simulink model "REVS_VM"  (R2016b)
settings: Solver=ode3  StartTime=REVS.sim_start_time_secs  StopTime=Inf  FixedStep=REVS.sim_step_time_secs  MaxStep=REVS.sim_step_time_secs  EnableMultiTasking=on
StopFcn:
  | postproc_datalog;
  | postproc_audit;
  | postproc_result;
model workspace (MATLAB code in the model file):
  other statements: REVS_setup_variants
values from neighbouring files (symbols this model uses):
  accessory = class_accessory_data    [class_test_data.m]
  battery = class_battery_data    [class_accessory_data.m]    (also in class_REVS_electric.m = class_REVS_battery)
  brake = struct(	'max_torque_Nm',[], 						'proportion_norm',1.0, 						'inertia_kgm2',0.0)    [class_REVS_drive_axle.m]
  engine = class_engine_data    [class_test_data.m]
  final_drive = struct(	'gear_ratio',[], 								'efficiency_norm',[], 								'inertia_kgm2',[] )    [class_REVS_drive_axle.m]
  gear = class_REVS_gearbox    [class_REVS_AT_transmission.m]
  tire = struct(	'radius_m',[], 						'rolling_resistance_coefficient',0, 						'vehicle_weight_norm',1.0,  						'wheel_slip_torque_Nm',[],  						'inertia_kgm2',0.0)    [class_REVS_drive_axle.m]
  torque_converter = class_REVS_torque_converter    [class_REVS_AT_transmission.m]
  transmission = class_transmission_data    [class_test_data.m]
  vehicle = class_vehicle_data    [class_test_data.m]
undefined symbols (not defined in the file or in its folder): alternator, ambient, controls, convert, DelayTimeSecs, drive_cycle, driver, electric, gear_strategy, InitialCondition, InitialValue, LoadSource, LookupStructure, MultiplyPosInputs, Normalize, NumPhases, REVS, SpeedSource, starter, tableshift, UpperSaturationLimit, Value, VerboseLevel, VerboseSignal
libraries: simulink x153
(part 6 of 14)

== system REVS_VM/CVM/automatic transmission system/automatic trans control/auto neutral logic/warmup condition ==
  bus : Inport
  Bus Creator : BusCreator  Inputs=10
  Bus Creator1 : BusCreator  Inputs=2
  Bus Selector : BusSelector  OutputSignals=var_sigs.var_sig1  OutputAsBus=on
  Data Type Conversion : DataTypeConversion  OutDataTypeStr=double
  Display : Display
  Fcn : Fcn
  Variable {1..10} (10 alike) : Constant  Value=nan
  out : Outport
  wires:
  Data Type Conversion/1 -> Fcn/1
  Bus Selector/1 -> Data Type Conversion/1, Display/1
  Bus Creator1/1 -> Bus Selector/1
  Fcn/1 -> out/1
  bus/1 -> Bus Creator1/1  "system_bus"
  Bus Creator/1 -> Bus Creator1/2  "var_sigs"
  Variable 1/1 -> Bus Creator/1  "var_sig1"
  Variable 2/1 -> Bus Creator/2  "var_sig2"
  Variable 3/1 -> Bus Creator/3  "var_sig3"
  Variable 4/1 -> Bus Creator/4  "var_sig4"
  Variable 5/1 -> Bus Creator/5  "var_sig5"
  Variable 6/1 -> Bus Creator/6  "var_sig6"
  Variable 7/1 -> Bus Creator/7  "var_sig7"
  Variable 8/1 -> Bus Creator/8  "var_sig8"
  Variable 9/1 -> Bus Creator/9  "var_sig9"
  Variable 10/1 -> Bus Creator/10  "var_sig10"

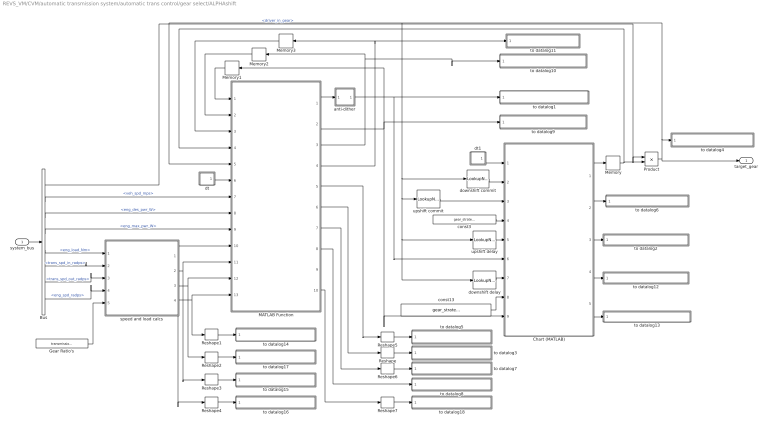
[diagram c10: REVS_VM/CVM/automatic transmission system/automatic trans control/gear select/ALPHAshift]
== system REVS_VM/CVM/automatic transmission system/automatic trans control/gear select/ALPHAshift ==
  system_bus : Inport
  Bus : BusSelector  OutputSignals=driver.driver_in_gear,vehicle.veh_spd_mps,powertrain.engine.eng_des_pwr_W,powertrain.engine.eng_max_pwr_W,powertrain.engine.eng_load_Nm,powertrain.trans.core.trans_spd_in_radps,powertrain.trans.core.trans_spd_out_radps,powertrain.engine.eng_spd_radps
  Chart (MATLAB) : Stateflow chart  TreatAsAtomicUnit=on
  Gear Ratio's : Constant  Value=transmission.gear.ratio  VectorParams1D=off
  MATLAB Function : MATLAB Function  TreatAsAtomicUnit=on
  Memory{,1..3} (4 alike) : Memory
  Product : Product
  Reshape{,1..7} (8 alike) : Reshape
  anti-dither : Subsystem
  const13 : Constant  Value=gear_strategy.disable_cost_saving_downshifts
  const3 : Constant  Value=gear_strategy.launch_gear_num
  downshift commit : LookupNDDirect  NumberOfTableDimensions=1  Table=gear_strategy.downshift_commit_secs
  downshift delay : LookupNDDirect  NumberOfTableDimensions=1  Table=gear_strategy.downshift_delay_secs
  dt : Subsystem
  dt1 : Subsystem
  speed and load calcs : Subsystem
  to datalog1 : Subsystem
  to datalog10 : Subsystem
  to datalog11 : Subsystem
  to datalog12 : Subsystem
  to datalog13 : Subsystem
  to datalog14 : Subsystem
  to datalog15 : Subsystem
  to datalog16 : Subsystem
  to datalog17 : Subsystem
  to datalog18 : Subsystem
  to datalog2 : Subsystem
  to datalog3 : Subsystem
  to datalog4 : Subsystem
  to datalog5 : Subsystem
  to datalog6 : Subsystem
  to datalog7 : Subsystem
  to datalog8 : Subsystem
  to datalog9 : Subsystem
  upshift commit : LookupNDDirect  NumberOfTableDimensions=1  Table=gear_strategy.upshift_commit_secs
  upshift delay : LookupNDDirect  NumberOfTableDimensions=1  Table=gear_strategy.upshift_delay_secs
  target_gear : Outport
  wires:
  MATLAB Function/10(kickdown_disability_code) -> Reshape7/1
  Reshape7/1 -> to datalog18/1(Var)
  Reshape2/1 -> to datalog17/1(Var)
  Chart (MATLAB)/5(in_gear_timer) -> to datalog13/1(Var)
  Chart (MATLAB)/4(shift_delay_timer) -> to datalog12/1(Var)
  speed and load calcs/1(gear_trq_Nm) -> Reshape4/1, MATLAB Function/10(gear_trq_Nm)
  Gear Ratio's/1 -> speed and load calcs/5(trans_gear_ratios)
  Bus/8 -> speed and load calcs/4(eng_spd_radps)  "<eng_spd_radps>"
  Bus/7 -> speed and load calcs/3(trans_spd_out_radps)  "<trans_spd_out_radps>"
  Bus/6 -> speed and load calcs/2(trans_spd_in_radps)  "<trans_spd_in_radps>"
  Bus/5 -> speed and load calcs/1(eng_load_Nm)  "<eng_load_Nm>"
  speed and load calcs/2(gear_spd_radps) -> Reshape3/1, MATLAB Function/11(gear_spd_radps)
  MATLAB Function/4(kickdown_ratio) -> to datalog11/1(Var), Memory3/1
  Memory3/1 -> MATLAB Function/3(kickdown_ratio_prev)
  Memory2/1 -> MATLAB Function/2(kickdown_timer_prev)
  MATLAB Function/3(kickdown_timer) -> Memory2/1, to datalog10/1(Var)
  Memory1/1 -> MATLAB Function/1(desired_shift_reason_prev)
  MATLAB Function/2(desired_shift_reason) -> to datalog9/1(Var), Memory1/1, Chart (MATLAB)/9(desired_shift_reason)
  const3/1 -> Chart (MATLAB)/4(launch_gear_num)
  const13/1 -> Chart (MATLAB)/8(legacy_downshift_mode)
  upshift delay/1 -> Chart (MATLAB)/5(upshift_delay_secs)
  downshift commit/1 -> Chart (MATLAB)/2(downshift_min_duration_secs)
  upshift commit/1 -> Chart (MATLAB)/3(upshift_min_duration_secs)
  downshift delay/1 -> Chart (MATLAB)/7(downshift_delay_secs)
  dt1/1(dt) -> Chart (MATLAB)/1(dt)
  Bus/1 -> Product/1  "<driver_in_gear>"
  Memory/1 -> MATLAB Function/4(command_gear_num), Product/2
  Bus/4 -> MATLAB Function/9(engine_max_pwr_W)  "<eng_max_pwr_W>"
  Bus/3 -> MATLAB Function/8(driver_des_pwr_W)  "<eng_des_pwr_W>"
  Chart (MATLAB)/2(previous_shift_type) -> to datalog6/1(Var)
  MATLAB Function/5(gear_available) -> Reshape5/1
  MATLAB Function/6(gear_disability_code) -> Reshape/1
  Chart (MATLAB)/3(shift_reason) -> to datalog2/1(Var)
  Product/1 -> MATLAB Function/5(current_gear_num), downshift commit/1, upshift commit/1, upshift delay/1, downshift delay/1, to datalog4/1(Var), target_gear/1
  system_bus/1 -> Bus/1
  speed and load calcs/3(gear_cost) -> MATLAB Function/12(gear_cost), Reshape2/1
  dt/1(dt) -> MATLAB Function/6(dt)
  Bus/2 -> MATLAB Function/7(vehicle_spd_mps)  "<veh_spd_mps>"
  Chart (MATLAB)/1(command_gear_num) -> Memory/1
  MATLAB Function/7(better_cost_gear) -> Reshape6/1
  MATLAB Function/8(min_cost_gear) -> to datalog8/1(Var)
  speed and load calcs/4(gear_avail_trq_Nm) -> Reshape1/1, MATLAB Function/13(gear_avail_trq_Nm)
  Reshape/1 -> to datalog3/1(Var)
  Reshape4/1 -> to datalog16/1(Var)
  Reshape3/1 -> to datalog15/1(Var)
  Reshape1/1 -> to datalog14/1(Var)
  anti-dither/1(out) -> to datalog1/1(Var), Chart (MATLAB)/6(desired_gear_num)
  MATLAB Function/1(desired_gear_num) -> anti-dither/1(raw)
  Reshape5/1 -> to datalog5/1(Var)
  Reshape6/1 -> to datalog7/1(Var)

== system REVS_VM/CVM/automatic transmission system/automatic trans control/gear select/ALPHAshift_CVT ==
  system_bus : Inport
  Bus Selector : BusSelector  OutputSignals=powertrain.trans.core.trans_spd_out_radps,driver.driver_in_gear,powertrain.engine.eng_des_pwr_W
  GR2SR : Fcn  Expr=1/u(1)
  MinMax : MinMax  Function=max  Inputs=2
  Product2 : Product  Inputs=**
  Product4 : Product  Inputs=*/
  SR Rate Limiter : RateLimiter  RisingSlewLimit=transmission.gear_strategy.speed_ratio_rise_rate_limit  FallingSlewLimit=-transmission.gear_strategy.speed_ratio_fall_rate_limit  SampleTimeMode=inherited
  SR2GR : Fcn  Expr=1/u(1)
  Saturation5 : Saturate  UpperLimit=max(transmission.gear.ratio)  LowerLimit=min(transmission.gear.ratio(2:end))
  eps : Saturate  UpperLimit=Inf  LowerLimit=eps
  min BSFC speed : Lookup_n-D  NumberOfTableDimensions=1  BreakpointsForDimension1=transmission.gear_strategy.min_bsfc_power_W  Table=transmission.gear_strategy.min_bsfc_speed_rapds  ExtrapMethod=Clip  InternalRulePriority=Speed  RndMeth=Simplest
  min speed table : Subsystem
  sat1 : Saturate  UpperLimit=2.48  LowerLimit=0.396
  sat2 : Saturate  UpperLimit=2.48  LowerLimit=0.396
  to datalog1 : Subsystem
  to datalog8 : Subsystem
  target_gear : Outport
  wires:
  MinMax/1 -> Product4/1, to datalog8/1(Var)
  min speed table/1(out) -> MinMax/2
  min BSFC speed/1 -> MinMax/1
  SR Rate Limiter/1 -> sat2/1
  Product2/1 -> GR2SR/1
  Bus Selector/2 -> Product2/1  "<driver_in_gear>"
  eps/1 -> Product4/2
  Saturation5/1 -> Product2/2
  Product4/1 -> Saturation5/1
  Bus Selector/3 -> min BSFC speed/1  "<eng_des_pwr_W>"
  Bus Selector/1 -> eps/1  "<trans_spd_out_radps>"
  system_bus/1 -> Bus Selector/1, min speed table/1(bus)
  SR2GR/1 -> target_gear/1, to datalog1/1(Var)
  sat2/1 -> SR2GR/1
  GR2SR/1 -> sat1/1
  sat1/1 -> SR Rate Limiter/1

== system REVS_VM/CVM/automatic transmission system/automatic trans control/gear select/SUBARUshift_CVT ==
  system_bus : Inport
  >= 1 : Saturate  UpperLimit=Inf  LowerLimit=1
  Bus Creator : BusCreator  Inputs=2
  Bus Creator1 : BusCreator  Inputs=2
  Bus Selector : BusSelector  OutputSignals=powertrain.trans.core.trans_spd_out_radps,driver.driver_in_gear
  Difference : simulink/Discrete/Difference  ICPrevInput=0.0  InputProcessing=Inherited  OutMin=[]  OutMax=[]  OutDataType=fixdt(1, 16)  OutScaling=2^-10  DoSatur=off
  Product : Product  Inputs=*/
  Product1 : Product  Inputs=*/
  Product2 : Product  Inputs=**
  Saturation : Saturate  UpperLimit=max(transmission.gear.ratio)  LowerLimit=min(transmission.gear.ratio(2:end))
  Saturation1 : Saturate  UpperLimit=max(transmission.gear.ratio)  LowerLimit=min(transmission.gear.ratio(2:end))
  Saturation2 : Saturate  UpperLimit=max(transmission.gear.ratio)  LowerLimit=min(transmission.gear.ratio(2:end))
  Switch : Switch  Criteria=u2 > Threshold
  downshift rate limit radps2 : Subsystem
  downshift time constant : Subsystem
  engine target radps : Subsystem
  eps : Saturate  UpperLimit=Inf  LowerLimit=eps
  target speed rate limiter : simulink/Discontinuities/Rate Limiter Dynamic
  upshift rate limit radps2 : Subsystem
  upshift time constant : Subsystem
  variable low pass filter : Subsystem
  target_gear : Outport
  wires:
  Product2/1 -> target_gear/1
  Saturation2/1 -> Product2/1  "cmd_ratio"
  Bus Selector/2 -> Product2/2  "<driver_in_gear>"
  engine target radps/1(out) -> >= 1/1
  variable low pass filter/1(out) -> Saturation2/1
  Switch/1 -> variable low pass filter/2(time const)
  Bus Creator1/1 -> downshift time constant/1(bus), upshift time constant/1(bus)
  upshift time constant/1(out) -> Switch/3
  downshift time constant/1(out) -> Switch/1
  Difference/1 -> Switch/2
  Saturation/1 -> variable low pass filter/1(in), Difference/1  "target_ratio"
  Bus Creator/1 -> downshift rate limit radps2/1(bus)
  Saturation1/1 -> Bus Creator/2  "desired_ratio"
  Product1/1 -> Saturation1/1
  >= 1/1 -> Product1/1, target speed rate limiter/2
  target speed rate limiter/1 -> Product/1, Bus Creator1/2  "desired_speed_radps"
  eps/1 -> Product1/2, Product/2
  upshift rate limit radps2/1(out) -> target speed rate limiter/3
  downshift rate limit radps2/1(out) -> target speed rate limiter/1
  Product/1 -> Saturation/1
  Bus Selector/1 -> eps/1  "<trans_spd_out_radps>"
  system_bus/1 -> upshift rate limit radps2/1(bus), Bus Selector/1, engine target radps/1(bus), Bus Creator/1, Bus Creator1/1

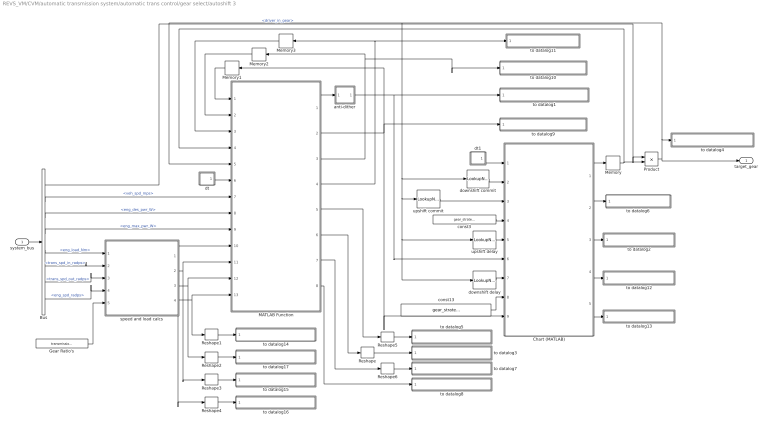
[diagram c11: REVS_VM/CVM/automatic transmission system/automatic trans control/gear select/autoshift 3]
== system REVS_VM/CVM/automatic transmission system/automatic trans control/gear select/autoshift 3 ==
  system_bus : Inport
  Bus : BusSelector  OutputSignals=driver.driver_in_gear,vehicle.veh_spd_mps,powertrain.engine.eng_des_pwr_W,powertrain.engine.eng_max_pwr_W,powertrain.engine.eng_load_Nm,powertrain.trans.core.trans_spd_in_radps,powertrain.trans.core.trans_spd_out_radps,powertrain.engine.eng_spd_radps
  Chart (MATLAB) : Stateflow chart  TreatAsAtomicUnit=on
  Gear Ratio's : Constant  Value=transmission.gear.ratio  VectorParams1D=off
  MATLAB Function : MATLAB Function  TreatAsAtomicUnit=on
  Memory{,1..3} (4 alike) : Memory
  Product : Product
  Reshape{,1..6} (7 alike) : Reshape
  anti-dither : Subsystem
  const13 : Constant  Value=gear_strategy.disable_cost_saving_downshifts
  const3 : Constant  Value=gear_strategy.launch_gear_num
  downshift commit : LookupNDDirect  NumberOfTableDimensions=1  Table=gear_strategy.downshift_commit_secs
  downshift delay : LookupNDDirect  NumberOfTableDimensions=1  Table=gear_strategy.downshift_delay_secs
  dt : Subsystem
  dt1 : Subsystem
  speed and load calcs : Subsystem
  to datalog1 : Subsystem
  to datalog10 : Subsystem
  to datalog11 : Subsystem
  to datalog12 : Subsystem
  to datalog13 : Subsystem
  to datalog14 : Subsystem
  to datalog15 : Subsystem
  to datalog16 : Subsystem
  to datalog17 : Subsystem
  to datalog2 : Subsystem
  to datalog3 : Subsystem
  to datalog4 : Subsystem
  to datalog5 : Subsystem
  to datalog6 : Subsystem
  to datalog7 : Subsystem
  to datalog8 : Subsystem
  to datalog9 : Subsystem
  upshift commit : LookupNDDirect  NumberOfTableDimensions=1  Table=gear_strategy.upshift_commit_secs
  upshift delay : LookupNDDirect  NumberOfTableDimensions=1  Table=gear_strategy.upshift_delay_secs
  target_gear : Outport
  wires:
  Reshape6/1 -> to datalog7/1(Var)
  Reshape5/1 -> to datalog5/1(Var)
  MATLAB Function/1(desired_gear_num) -> anti-dither/1(raw)
  anti-dither/1(out) -> to datalog1/1(Var), Chart (MATLAB)/6(desired_gear_num)
  Reshape1/1 -> to datalog14/1(Var)
  Reshape3/1 -> to datalog15/1(Var)
  Reshape4/1 -> to datalog16/1(Var)
  Reshape/1 -> to datalog3/1(Var)
  speed and load calcs/4(gear_avail_trq_Nm) -> MATLAB Function/13(gear_avail_trq_Nm), Reshape1/1
  MATLAB Function/8(min_cost_gear) -> to datalog8/1(Var)
  MATLAB Function/7(better_cost_gear) -> Reshape6/1
  Chart (MATLAB)/1(command_gear_num) -> Memory/1
  Bus/2 -> MATLAB Function/7(vehicle_spd_mps)  "<veh_spd_mps>"
  dt/1(dt) -> MATLAB Function/6(dt)
  speed and load calcs/3(gear_cost) -> Reshape2/1, MATLAB Function/12(gear_cost)
  system_bus/1 -> Bus/1
  Product/1 -> target_gear/1, to datalog4/1(Var), downshift delay/1, upshift delay/1, upshift commit/1, downshift commit/1, MATLAB Function/5(current_gear_num)
  Chart (MATLAB)/3(shift_reason) -> to datalog2/1(Var)
  MATLAB Function/6(gear_disability_code) -> Reshape/1
  MATLAB Function/5(gear_available) -> Reshape5/1
  Chart (MATLAB)/2(previous_shift_type) -> to datalog6/1(Var)
  Bus/3 -> MATLAB Function/8(driver_des_pwr_W)  "<eng_des_pwr_W>"
  Bus/4 -> MATLAB Function/9(engine_max_pwr_W)  "<eng_max_pwr_W>"
  Memory/1 -> Product/2, MATLAB Function/4(command_gear_num)
  Bus/1 -> Product/1  "<driver_in_gear>"
  dt1/1(dt) -> Chart (MATLAB)/1(dt)
  downshift delay/1 -> Chart (MATLAB)/7(downshift_delay_secs)
  upshift commit/1 -> Chart (MATLAB)/3(upshift_min_duration_secs)
  downshift commit/1 -> Chart (MATLAB)/2(downshift_min_duration_secs)
  upshift delay/1 -> Chart (MATLAB)/5(upshift_delay_secs)
  const13/1 -> Chart (MATLAB)/8(legacy_downshift_mode)
  const3/1 -> Chart (MATLAB)/4(launch_gear_num)
  MATLAB Function/2(desired_shift_reason) -> Memory1/1, Chart (MATLAB)/9(desired_shift_reason), to datalog9/1(Var)
  Memory1/1 -> MATLAB Function/1(desired_shift_reason_prev)
  MATLAB Function/3(kickdown_timer) -> to datalog10/1(Var), Memory2/1
  Memory2/1 -> MATLAB Function/2(kickdown_timer_prev)
  Memory3/1 -> MATLAB Function/3(kickdown_ratio_prev)
  MATLAB Function/4(kickdown_ratio) -> Memory3/1, to datalog11/1(Var)
  speed and load calcs/2(gear_spd_radps) -> MATLAB Function/11(gear_spd_radps), Reshape3/1
  Bus/5 -> speed and load calcs/1(eng_load_Nm)  "<eng_load_Nm>"
  Bus/6 -> speed and load calcs/2(trans_spd_in_radps)  "<trans_spd_in_radps>"
  Bus/7 -> speed and load calcs/3(trans_spd_out_radps)  "<trans_spd_out_radps>"
  Bus/8 -> speed and load calcs/4(eng_spd_radps)  "<eng_spd_radps>"
  Gear Ratio's/1 -> speed and load calcs/5(trans_gear_ratios)
  speed and load calcs/1(gear_trq_Nm) -> MATLAB Function/10(gear_trq_Nm), Reshape4/1
  Chart (MATLAB)/4(shift_delay_timer) -> to datalog12/1(Var)
  Chart (MATLAB)/5(in_gear_timer) -> to datalog13/1(Var)
  Reshape2/1 -> to datalog17/1(Var)

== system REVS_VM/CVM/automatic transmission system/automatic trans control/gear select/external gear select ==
  system_bus : Inport
  Bus Selector : BusSelector  OutputSignals=driver.cycle_pos_secs
  drive cycle : Lookup_n-D  NumberOfTableDimensions=1  BreakpointsForDimension1=transmission.gear_strategy.time_secs  IndexSearchMethod=Linear search  BeginIndexSearchUsingPreviousIndexResult=on  Table=transmission.gear_strategy.gear_num  InterpMethod=Flat  ExtrapMethod=Clip  UseLastTableValue=on  RndMeth=Simplest  MaximumIndicesForEachDimension=1e5
  target_gear : Outport
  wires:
  system_bus/1 -> Bus Selector/1
  Bus Selector/1 -> drive cycle/1  "<cycle_pos_secs>"
  drive cycle/1 -> target_gear/1

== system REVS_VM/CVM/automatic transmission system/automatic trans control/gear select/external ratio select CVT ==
  system_bus : Inport
  Bus Selector : BusSelector  OutputSignals=driver.cycle_pos_secs,driver.driver_in_gear
  CVT ratio : Lookup_n-D  NumberOfTableDimensions=1  BreakpointsForDimension1=gear_strategy.time_secs  IndexSearchMethod=Linear search  BeginIndexSearchUsingPreviousIndexResult=on  Table=gear_strategy.CVT_ratio  ExtrapMethod=Clip  UseLastTableValue=on  RndMeth=Simplest  MaximumIndicesForEachDimension=1e5
  Product2 : Product  Inputs=**
  Saturation3 : Saturate  UpperLimit=max(transmission.gear.ratio)  LowerLimit=min(transmission.gear.ratio(2:end))
  target_gear : Outport
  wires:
  Product2/1 -> target_gear/1
  Saturation3/1 -> Product2/1
  CVT ratio/1 -> Saturation3/1
  Bus Selector/1 -> CVT ratio/1  "<cycle_pos_secs>"
  system_bus/1 -> Bus Selector/1
  Bus Selector/2 -> Product2/2  "<driver_in_gear>"

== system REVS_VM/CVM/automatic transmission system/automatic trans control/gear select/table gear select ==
  system_bus : Inport
  Bus Selector : BusSelector  OutputSignals=driver.driver_in_gear
  Downshift : Lookup_n-D  BreakpointsForDimension1=tableshift.downshift_map_load  BreakpointsForDimension2=(1:size(tableshift.downshift_map_speed,2))-1  IndexSearchMethod=Linear search  BeginIndexSearchUsingPreviousIndexResult=on  Table=tableshift.downshift_map_speed  ExtrapMethod=Clip  DiagnosticForOutOfRangeInput=Error  UseLastTableValue=on  RndMeth=Simplest
  Downshift Delay : LookupNDDirect  NumberOfTableDimensions=1  Table=tableshift.downshift_delay_secs  DiagnosticForOutOfRangeInput=Error
  Memory1 : Memory  X0=1
  Product : Product
  Saturation : Saturate  UpperLimit=transmission.gear.number(end)  LowerLimit=0  ZeroCross=off
  Upshift : Lookup_n-D  BreakpointsForDimension1=tableshift.upshift_map_load  BreakpointsForDimension2=(1:size(tableshift.upshift_map_speed,2))-1  IndexSearchMethod=Linear search  BeginIndexSearchUsingPreviousIndexResult=on  Table=tableshift.upshift_map_speed  ExtrapMethod=Clip  DiagnosticForOutOfRangeInput=Error  UseLastTableValue=on  RndMeth=Simplest
  Upshift Delay : LookupNDDirect  NumberOfTableDimensions=1  Table=tableshift.upshift_delay_secs  DiagnosticForOutOfRangeInput=Error
  dt : Subsystem
  gear shifting : Stateflow chart  TreatAsAtomicUnit=on
  shift load select : Subsystem
  shift speed select : Subsystem
  target_gear : Outport
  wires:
  Saturation/1 -> target_gear/1
  Downshift Delay/1 -> gear shifting/6(downshift_delay_secs)
  Bus Selector/1 -> Product/2  "<driver_in_gear>"
  Product/1 -> Saturation/1
  shift speed select/1(spd) -> gear shifting/1(shift_spd)
  Downshift/1 -> gear shifting/5(downshift_spd)
  shift load select/1(load) -> Upshift/1, Downshift/1
  Upshift/1 -> gear shifting/4(upshift_spd)
  Upshift Delay/1 -> gear shifting/3(upshift_delay_secs)
  Memory1/1 -> Downshift Delay/1, Downshift/2, Upshift Delay/1, Upshift/2
  gear shifting/1(driver_gear) -> Memory1/1, Product/1
  system_bus/1 -> Bus Selector/1, shift speed select/1(system_bus), shift load select/1(system_bus)
  dt/1(dt) -> gear shifting/2(step_time)

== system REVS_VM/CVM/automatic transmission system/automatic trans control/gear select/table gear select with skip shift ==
  system_bus : Inport
  Bus Selector : BusSelector  OutputSignals=driver.driver_in_gear
  Compare To Constant : simulink/Logic and Bit Operations/Compare To Constant  relop=>  const=3.0  OutDataTypeStr=boolean  ZeroCross=off
  Constant : Constant
  Constant1 : Constant
  Down Shift Timer : Subsystem
  Downshift : Lookup_n-D  BreakpointsForDimension1=tableshift.downshift_map_load  BreakpointsForDimension2=(1:size(tableshift.downshift_map_speed,2))-1  IndexSearchMethod=Linear search  BeginIndexSearchUsingPreviousIndexResult=on  Table=tableshift.downshift_map_speed  ExtrapMethod=Clip  UseLastTableValue=on  RndMeth=Simplest
  Downshift Delay : LookupNDDirect  NumberOfTableDimensions=1  Table=tableshift.downshift_delay_secs
  Downshift Skip Pedal : LookupNDDirect  NumberOfTableDimensions=1  Table=tableshift.downshift_skip_pedal_pct
  Downshift Switch : Switch  Criteria=u2 ~= 0
  Logical Operator : Logic  AllPortsSameDT=off  OutDataTypeStr=boolean
  Memory4 : Memory  X0=1
  Product : Product
  Relational Operator : RelationalOperator  Operator=>  OutDataTypeStr=boolean  ZeroCross=off
  Relational Operator1 : RelationalOperator  Operator=<  OutDataTypeStr=boolean  ZeroCross=off
  Relational Operator2 : RelationalOperator  OutDataTypeStr=boolean  ZeroCross=off
  Relational Operator3 : RelationalOperator  Operator=>  OutDataTypeStr=boolean  ZeroCross=off
  Relational Operator4 : RelationalOperator  Operator=<=  OutDataTypeStr=boolean  ZeroCross=off
  Relational Operator5 : RelationalOperator  Operator=>  OutDataTypeStr=boolean  ZeroCross=off
  Saturation : Saturate  UpperLimit=inf  LowerLimit=1  ZeroCross=off
  Sum : Sum  Inputs=+++
  Sum1 : Sum  Inputs=+--
  Time Since Upshift : Subsystem
  Up Shift Timer : Subsystem
  Upshift : Lookup_n-D  BreakpointsForDimension1=tableshift.upshift_map_load  BreakpointsForDimension2=(1:size(tableshift.upshift_map_speed,2))-1  IndexSearchMethod=Linear search  BeginIndexSearchUsingPreviousIndexResult=on  Table=tableshift.upshift_map_speed  ExtrapMethod=Clip  UseLastTableValue=on  RndMeth=Simplest
  Upshift Delay : LookupNDDirect  NumberOfTableDimensions=1  Table=tableshift.upshift_delay_secs
  Upshift Skip Pedal : LookupNDDirect  NumberOfTableDimensions=1  Table=tableshift.upshift_skip_pedal_pct
  Upshift Switch : Switch  Criteria=u2 ~= 0
  load select : Subsystem
  speed select : Subsystem
  target_gear : Outport
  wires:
  Product/1 -> target_gear/1
  Bus Selector/1 -> Product/1  "<driver_in_gear>"
  system_bus/1 -> speed select/1(system_bus), load select/1(system_bus), Bus Selector/1
  Downshift Switch/1 -> Saturation/1
  Upshift Delay/1 -> Relational Operator3/2
  Upshift/1 -> Relational Operator/2
  load select/1(load) -> Upshift/1, Relational Operator2/1, Relational Operator4/1, Downshift/1
  Downshift/1 -> Relational Operator1/2
  speed select/1(spd) -> Relational Operator/1, Relational Operator1/1
  Relational Operator/1 -> Up Shift Timer/1(Bool)
  Relational Operator1/1 -> Down Shift Timer/1(Bool)
  Memory4/1 -> Upshift Skip Pedal/1, Upshift Delay/1, Upshift/2, Sum/3, Sum1/1, Downshift Skip Pedal/1, Downshift/2, Downshift Delay/1, Upshift Switch/3
  Downshift Delay/1 -> Relational Operator5/2
  Down Shift Timer/1(Timer) -> Relational Operator5/1
  Up Shift Timer/1(Timer) -> Relational Operator3/1
  Relational Operator3/1 -> Time Since Upshift/1(Bool), Upshift Switch/2
  Upshift Switch/1 -> Downshift Switch/3
  Relational Operator5/1 -> Logical Operator/2
  Upshift Skip Pedal/1 -> Relational Operator2/2
  Relational Operator2/1 -> Sum/2
  Constant/1 -> Sum/1
  Sum/1 -> Upshift Switch/1
  Constant1/1 -> Sum1/3
  Sum1/1 -> Downshift Switch/1
  Downshift Skip Pedal/1 -> Relational Operator4/2
  Relational Operator4/1 -> Sum1/2
  Saturation/1 -> Memory4/1, Product/2
  Logical Operator/1 -> Downshift Switch/2
  Time Since Upshift/1(Timer) -> Compare To Constant/1
  Compare To Constant/1 -> Logical Operator/1

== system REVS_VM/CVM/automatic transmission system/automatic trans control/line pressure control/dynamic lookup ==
  bus : Inport
  Bus Selector : BusSelector  OutputSignals=gb.gb_cmd_gear,gb_spd_in_radps,ctrl.gb_line_press_bar
  Lookup : Lookup_n-D  NumberOfTableDimensions=10  BreakpointsForDimension1=LookupStructure.axis_1.breakpoints  BreakpointsForDimension2=LookupStructure.axis_2.breakpoints  BreakpointsForDimension3=LookupStructure.axis_3.breakpoints  BreakpointsForDimension4=LookupStructure.axis_4.breakpoints  BreakpointsForDimension5=LookupStructure.axis_5.breakpoints  BreakpointsForDimension6=LookupStructure.axis_6.breakpoints  BreakpointsForDimension7=LookupStructure.axis_7.breakpoints  BreakpointsForDimension8=LookupStructure.axis_8.breakpoints  BreakpointsForDimension9=LookupStructure.axis_9.breakpoints  BreakpointsForDimension10=LookupStructure.axis_10.breakpoints  IndexSearchMethod=Linear search  BeginIndexSearchUsingPreviousIndexResult=on  Table=LookupStructure.table  DiagnosticForOutOfRangeInput=Warning  InternalRulePriority=Speed  RndMeth=Simplest  SupportTunableTableSize=on  MaximumIndicesForEachDimension=LookupStructure.table_size
  out : Outport
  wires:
  bus/1 -> Bus Selector/1
  Lookup/1 -> out/1

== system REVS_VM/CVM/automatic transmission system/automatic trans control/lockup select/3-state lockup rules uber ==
  gear_number : Inport
  system_bus : Inport  Port=2
  Bus Selector : BusSelector  OutputSignals=powertrain.trans.ctrl.gear_num
  Constant : Constant  Value=inf
  Constant1 : Constant  Value=transmission.tcc_strategy.upshift_slip_speed_radps
  Detect Decrease1 : simulink/Logic and Bit Operations/Detect Decrease  vinit=0.0  InputProcessing=Inherited  OutDataTypeStr=boolean
  Detect Increase1 : simulink/Logic and Bit Operations/Detect Increase  vinit=0.0  InputProcessing=Inherited  OutDataTypeStr=boolean
  MinMax : MinMax  Function=max  Inputs=3  ZeroCross=off
  Product : Product
  Product1 : Product
  Product2 : Product
  Rate Limiter : RateLimiter  RisingSlewLimit=transmission.tcc_strategy.disengage_rate_radps2  FallingSlewLimit=-transmission.tcc_strategy.engage_rate_radps2  InitialCondition=100
  Relay : Relay  OnSwitchValue=transmission.tcc_strategy.lockup_hysteresis_radps * 1.5  OffSwitchValue=transmission.tcc_strategy.lockup_hysteresis_radps * 0.5  ZeroCross=off
  Saturation : Saturate  UpperLimit=1000 * convert.rpm2radps  LowerLimit=0  ZeroCross=off
  Switch : Switch  Criteria=u2 > Threshold  Threshold=1000 * convert.rpm2radps
  downshift slip speed : Constant  Value=transmission.tcc_strategy.downshift_slip_speed_radps
  downshift timer : Subsystem
  target slip table : Subsystem
  upshift timer : Subsystem
  lockup_cmd : Outport
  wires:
  target slip table/1(out) -> Product2/2, Relay/1
  Relay/1 -> Product2/1
  Switch/1 -> lockup_cmd/1
  Saturation/1 -> Rate Limiter/1
  MinMax/1 -> Saturation/1, Switch/2
  Product1/1 -> MinMax/3
  Product/1 -> MinMax/2
  Constant1/1 -> Product1/2
  downshift slip speed/1 -> Product/2
  upshift timer/1(timer_bool) -> Product1/1
  Detect Increase1/1 -> upshift timer/1(trigger_bool)
  downshift timer/1(timer_bool) -> Product/1
  Detect Decrease1/1 -> downshift timer/1(trigger_bool)
  Product2/1 -> MinMax/1
  system_bus/1 -> Bus Selector/1, target slip table/1(bus)
  Bus Selector/1 -> Detect Decrease1/1, Detect Increase1/1  "<gear_num>"
  Rate Limiter/1 -> Switch/3
  Constant/1 -> Switch/1

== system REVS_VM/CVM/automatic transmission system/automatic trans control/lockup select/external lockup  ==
  gear_number : Inport
  system_bus : Inport  Port=2
  1-D Lookup Table : Lookup_n-D  NumberOfTableDimensions=1  BreakpointsForDimension1=transmission.tcc_strategy.time_sec  IndexSearchMethod=Linear search  BeginIndexSearchUsingPreviousIndexResult=on  Table=transmission.tcc_strategy.lock_up  InterpMethod=Flat  ExtrapMethod=Clip  InternalRulePriority=Speed  RndMeth=Simplest
  Bus Selector : BusSelector  OutputSignals=driver.cycle_pos_secs
  lockup_cmd : Outport
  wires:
  1-D Lookup Table/1 -> lockup_cmd/1  "tcc_lock_up_cmd"
  system_bus/1 -> Bus Selector/1
  Bus Selector/1 -> 1-D Lookup Table/1  "<cycle_pos_secs>"

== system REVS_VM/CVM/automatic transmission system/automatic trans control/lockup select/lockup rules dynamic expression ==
  gear_number : Inport
  system_bus : Inport  Port=2
  Compare To Constant : simulink/Logic and Bit Operations/Compare To Constant  relop=>=  const=transmission.torque_converter.always_lock_gear  OutDataTypeStr=boolean  ZeroCross=off
  Compare To Constant6 : simulink/Logic and Bit Operations/Compare To Constant  relop=>  const=transmission.torque_converter.always_unlock_gear  OutDataTypeStr=boolean  ZeroCross=off
  Data Type Conversion : DataTypeConversion
  Detect Decrease : simulink/Logic and Bit Operations/Detect Decrease  vinit=0.0  InputProcessing=Inherited  OutDataTypeStr=boolean
  Detect Increase : simulink/Logic and Bit Operations/Detect Increase  vinit=0.0  InputProcessing=Inherited  OutDataTypeStr=boolean
  Logical Operator1 : Logic  AllPortsSameDT=off  OutDataTypeStr=boolean
  Logical Operator2 : Logic  Operator=NAND  AllPortsSameDT=off  OutDataTypeStr=boolean
  Logical Operator3 : Logic  Operator=NOT  AllPortsSameDT=off  OutDataTypeStr=boolean
  Logical Operator6 : Logic  Operator=NAND  AllPortsSameDT=off  OutDataTypeStr=boolean
  Logical Operator8 : Logic  Operator=OR  Inputs=3  AllPortsSameDT=off  OutDataTypeStr=boolean
  Logical Operator9 : Logic  Inputs=5  AllPortsSameDT=off  OutDataTypeStr=boolean
  Memory : Memory
  Relational Operator : RelationalOperator  Operator=>  OutDataTypeStr=boolean  ZeroCross=off
  boolean integrator : Subsystem
  const1 : Constant  Value=transmission.torque_converter.lockup_allowed
  const3 : Constant  Value=transmission.torque_converter.lockup_delay_secs
  downshift unlock criteria : Subsystem
  lockup equation : Subsystem
  unlock equation : Subsystem
  upshift unlock criteria : Subsystem
  lockup_cmd : Outport
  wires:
  Memory/1 -> Logical Operator1/2
  Logical Operator3/1 -> Logical Operator1/1
  Logical Operator1/1 -> Logical Operator8/3
  upshift unlock criteria/1(out) -> Logical Operator2/1
  downshift unlock criteria/1(out) -> Logical Operator6/1
  unlock equation/1(out) -> Logical Operator3/1
  Compare To Constant/1 -> Logical Operator8/1
  Data Type Conversion/1 -> lockup_cmd/1, Memory/1  "tcc_lockup_cmd_bool"
  Relational Operator/1 -> Data Type Conversion/1
  const1/1 -> Logical Operator9/1
  boolean integrator/1(out) -> Relational Operator/1
  gear_number/1 -> Detect Decrease/1, Detect Increase/1, Compare To Constant/1, Compare To Constant6/1
  lockup equation/1(out) -> Logical Operator8/2
  Detect Decrease/1 -> Logical Operator6/2
  const3/1 -> Relational Operator/2
  Compare To Constant6/1 -> Logical Operator9/2
  Logical Operator8/1 -> Logical Operator9/5
  Logical Operator9/1 -> boolean integrator/1(bool)
  system_bus/1 -> lockup equation/1(bus), downshift unlock criteria/1(bus), upshift unlock criteria/1(bus), unlock equation/1(bus)
  Detect Increase/1 -> Logical Operator2/2
  Logical Operator2/1 -> Logical Operator9/4
  Logical Operator6/1 -> Logical Operator9/3

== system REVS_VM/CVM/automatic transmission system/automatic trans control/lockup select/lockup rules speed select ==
  gear_number : Inport
  system_bus : Inport  Port=2
  Compare To Constant : simulink/Logic and Bit Operations/Compare To Constant  relop=>=  const=transmission.torque_converter.always_lock_gear  OutDataTypeStr=boolean  ZeroCross=off
  Compare To Constant1 : simulink/Logic and Bit Operations/Compare To Constant  relop=>  const=transmission.torque_converter.lockup_speed  OutDataTypeStr=boolean  ZeroCross=off
  Compare To Constant2 : simulink/Logic and Bit Operations/Compare To Constant  relop=<  const=transmission.torque_converter.unlock_speed  OutDataTypeStr=boolean  ZeroCross=off
  Compare To Constant6 : simulink/Logic and Bit Operations/Compare To Constant  relop=>  const=transmission.torque_converter.always_unlock_gear  OutDataTypeStr=boolean  ZeroCross=off
  Data Type Conversion : DataTypeConversion
  Detect Decrease : simulink/Logic and Bit Operations/Detect Decrease  vinit=0.0  InputProcessing=Inherited  OutDataTypeStr=boolean
  Detect Increase : simulink/Logic and Bit Operations/Detect Increase  vinit=0.0  InputProcessing=Inherited  OutDataTypeStr=boolean
  Latch : Subsystem
  Logical Operator2 : Logic  Operator=NAND  AllPortsSameDT=off  OutDataTypeStr=boolean
  Logical Operator6 : Logic  Operator=NAND  AllPortsSameDT=off  OutDataTypeStr=boolean
  Logical Operator8 : Logic  Operator=OR  AllPortsSameDT=off  OutDataTypeStr=boolean
  Logical Operator9 : Logic  Inputs=5  AllPortsSameDT=off  OutDataTypeStr=boolean
  Relational Operator : RelationalOperator  Operator=>  OutDataTypeStr=boolean  ZeroCross=off
  boolean integrator : Subsystem
  const1 : Constant  Value=transmission.torque_converter.lockup_allowed
  const2 : Constant  Value=transmission.torque_converter.unlock_downshift_bool
  const3 : Constant  Value=transmission.torque_converter.lockup_delay_secs
  const4 : Constant  Value=transmission.torque_converter.unlock_upshift_bool
  lockup speed select : Subsystem
  lockup_cmd : Outport
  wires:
  lockup speed select/1(spd) -> Compare To Constant1/1, Compare To Constant2/1
  Compare To Constant2/1 -> Latch/2(Off)
  Compare To Constant/1 -> Logical Operator8/1
  Data Type Conversion/1 -> lockup_cmd/1  "tcc_lockup_cmd_bool"
  Relational Operator/1 -> Data Type Conversion/1
  const1/1 -> Logical Operator9/1
  boolean integrator/1(out) -> Relational Operator/1
  gear_number/1 -> Detect Increase/1, Compare To Constant/1, Detect Decrease/1, Compare To Constant6/1
  Latch/1(State) -> Logical Operator8/2
  Compare To Constant1/1 -> Latch/1(On)
  Detect Decrease/1 -> Logical Operator6/2
  const3/1 -> Relational Operator/2
  const2/1 -> Logical Operator6/1
  Compare To Constant6/1 -> Logical Operator9/2
  Logical Operator8/1 -> Logical Operator9/5
  Logical Operator9/1 -> boolean integrator/1(bool)
  system_bus/1 -> lockup speed select/1(system_bus)
  const4/1 -> Logical Operator2/1
  Detect Increase/1 -> Logical Operator2/2
  Logical Operator2/1 -> Logical Operator9/4
  Logical Operator6/1 -> Logical Operator9/3

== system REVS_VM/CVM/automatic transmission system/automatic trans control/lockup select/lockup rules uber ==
  gear_number : Inport
  system_bus : Inport  Port=2
  Bus Creator1 : BusCreator  Inputs=3
  Data Type Conversion : DataTypeConversion
  Detect Decrease : simulink/Logic and Bit Operations/Detect Decrease  vinit=0.0  InputProcessing=Inherited  OutDataTypeStr=boolean
  Detect Increase : simulink/Logic and Bit Operations/Detect Increase  vinit=0.0  InputProcessing=Inherited  OutDataTypeStr=boolean
  Logical Operator2 : Logic  Operator=NAND  AllPortsSameDT=off  OutDataTypeStr=boolean
  Logical Operator3 : Logic  Operator=NOT  AllPortsSameDT=off  OutDataTypeStr=boolean
  Logical Operator6 : Logic  Operator=NAND  AllPortsSameDT=off  OutDataTypeStr=boolean
  Logical Operator8 : Logic  Operator=OR  AllPortsSameDT=off  OutDataTypeStr=boolean
  Logical Operator9 : Logic  Inputs=5  AllPortsSameDT=off  OutDataTypeStr=boolean
  Memory : Memory
  Relational Operator : RelationalOperator  Operator=>  OutDataTypeStr=boolean  ZeroCross=off
  boolean integrator : Subsystem
  const1 : Constant  Value=transmission.tcc_strategy.lockup_allowed
  const3 : Constant  Value=transmission.tcc_strategy.lockup_delay_secs
  downshift unlock criteria : Subsystem
  lockup criteria : Subsystem
  lockup table : Subsystem
  unlock criteria : Subsystem
  unlock table : Subsystem
  upshift unlock criteria : Subsystem
  lockup_cmd : Outport
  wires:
  Memory/1 -> Logical Operator8/1
  lockup criteria/1(out) -> Logical Operator8/2
  unlock table/1(out) -> Bus Creator1/2  "table_unlock_spd"
  Bus Creator1/1 -> unlock criteria/1(bus), lockup criteria/1(bus)
  lockup table/1(out) -> Bus Creator1/1  "table_lock_spd"
  Logical Operator3/1 -> Logical Operator9/5
  upshift unlock criteria/1(out) -> Logical Operator2/1
  downshift unlock criteria/1(out) -> Logical Operator6/1
  unlock criteria/1(out) -> Logical Operator3/1
  Data Type Conversion/1 -> Memory/1, lockup_cmd/1  "tcc_lockup_cmd_bool"
  Relational Operator/1 -> Data Type Conversion/1
  const1/1 -> Logical Operator9/1
  boolean integrator/1(out) -> Relational Operator/1
  gear_number/1 -> Detect Decrease/1, Detect Increase/1
  Detect Decrease/1 -> Logical Operator6/2
  const3/1 -> Relational Operator/2
  Logical Operator8/1 -> Logical Operator9/4
  Logical Operator9/1 -> boolean integrator/1(bool)
  system_bus/1 -> downshift unlock criteria/1(bus), upshift unlock criteria/1(bus), lockup table/1(bus), unlock table/1(bus), Bus Creator1/3  "system_bus"
  Detect Increase/1 -> Logical Operator2/2
  Logical Operator2/1 -> Logical Operator9/3
  Logical Operator6/1 -> Logical Operator9/2

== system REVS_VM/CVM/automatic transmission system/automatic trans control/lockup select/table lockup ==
  gear_number : Inport
  system_bus : Inport  Port=2
  const : Constant  Value=transmission.tcc_strategy.lockup_allowed
  const2 : Constant  Value=transmission.tcc_strategy.lockup_delay_secs
  dt : Subsystem
  "lock map " : Lookup_n-D  BreakpointsForDimension1=transmission.tcc_strategy.lock_map_load  BreakpointsForDimension2=transmission.gear.number(2:end)  Table=transmission.tcc_strategy.lock_map_speed  RndMeth=Simplest
  lockup load select : Subsystem
  lockup speed select : Subsystem
  tcc lockup : Stateflow chart  TreatAsAtomicUnit=on
  "unlock map " : Lookup_n-D  BreakpointsForDimension1=transmission.tcc_strategy.unlock_map_load  BreakpointsForDimension2=transmission.gear.number(2:end)  Table=transmission.tcc_strategy.unlock_map_speed  RndMeth=Simplest
  lockup_cmd : Outport
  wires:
  gear_number/1 -> "unlock map "/2, "lock map "/2
  system_bus/1 -> lockup speed select/1(system_bus), lockup load select/1(system_bus)
  const2/1 -> tcc lockup/6(lockup_delay_secs)
  lockup load select/1(load) -> "lock map "/1, "unlock map "/1
  const/1 -> tcc lockup/5(lockup_allowed)
  tcc lockup/1(tcc_lockup) -> lockup_cmd/1  "tcc_lockup_cmd_bool"
  "lock map "/1 -> tcc lockup/3(lockup_spd)
  "unlock map "/1 -> tcc lockup/4(release_spd)
  lockup speed select/1(spd) -> tcc lockup/1(lock_spd)
  dt/1(dt) -> tcc lockup/2(step_time)

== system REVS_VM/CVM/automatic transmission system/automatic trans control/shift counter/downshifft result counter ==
  in : Inport
  Data Type Conversion : DataTypeConversion  OutDataTypeStr=double
  Phase Memory : Memory
  Phase To Workspace : ToWorkspace  VariableName=result__phase_num_downshifts  SampleTime=-1
  Product : Product
  Sum : Sum  Inputs=|++
  Sum1 : Sum  Inputs=|++
  Total Memory : Memory
  Total To Workspace : ToWorkspace  VariableName=result__total_num_downshifts  SampleTime=-1
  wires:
  Data Type Conversion/1 -> Product/2, Sum1/1
  Sum1/1 -> Total Memory/1
  Sum/1 -> Phase Memory/1
  in/1 -> Data Type Conversion/1
  Total Memory/1 -> Sum1/2, Total To Workspace/1
  Product/1 -> Sum/1
  [REVS_phase_flag] -> Product/1
  Phase Memory/1 -> Phase To Workspace/1, Sum/2

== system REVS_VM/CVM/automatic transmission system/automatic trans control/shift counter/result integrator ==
  in : Inport
  Data Type Conversion : DataTypeConversion  OutDataTypeStr=double
  Integrator1 : Integrator  UpperSaturationLimit=Inf  LowerSaturationLimit=0  ZeroCross=off
  Integrator2 : Integrator  UpperSaturationLimit=Inf  LowerSaturationLimit=0  ZeroCross=off
  Phase To Workspace : ToWorkspace  VariableName=result__phase_gear_time_secs  SampleTime=-1
  Product1 : Product  Multiplication=Matrix(*)
  Reshape : Reshape
  Total To Workspace : ToWorkspace  VariableName=result__total_gear_time_secs  SampleTime=-1
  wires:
  Reshape/1 -> Integrator1/1, Product1/1
  Data Type Conversion/1 -> Reshape/1
  Integrator2/1 -> Phase To Workspace/1
  [REVS_phase_flag] -> Product1/2
  Product1/1 -> Integrator2/1
  Integrator1/1 -> Total To Workspace/1
  in/1 -> Data Type Conversion/1

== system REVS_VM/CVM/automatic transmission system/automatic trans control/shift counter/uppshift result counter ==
  in : Inport
  Data Type Conversion : DataTypeConversion  OutDataTypeStr=double
  Phase Memory : Memory
  Phase To Workspace : ToWorkspace  VariableName=result__phase_num_upshifts  SampleTime=-1
  Product : Product
  Sum : Sum  Inputs=|++
  Sum1 : Sum  Inputs=|++
  Total Memory : Memory
  Total To Workspace : ToWorkspace  VariableName=result__total_num_upshifts  SampleTime=-1
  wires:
  Data Type Conversion/1 -> Product/2, Sum1/1
  Sum1/1 -> Total Memory/1
  Sum/1 -> Phase Memory/1
  in/1 -> Data Type Conversion/1
  Total Memory/1 -> Sum1/2, Total To Workspace/1
  Product/1 -> Sum/1
  [REVS_phase_flag] -> Product/1
  Phase Memory/1 -> Phase To Workspace/1, Sum/2

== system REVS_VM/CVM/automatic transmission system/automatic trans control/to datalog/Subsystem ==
  In1 : Inport
  Enable : EnablePort
  To Workspace : ToWorkspace  VariableName=datalog__transmission__torque_converter_clutch_command_norm  SampleTime=-1
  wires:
  In1/1 -> To Workspace/1

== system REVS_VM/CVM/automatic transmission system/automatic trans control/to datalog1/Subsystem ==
  In1 : Inport
  Enable : EnablePort
  To Workspace : ToWorkspace  VariableName=datalog__transmission__selected_gear_num  SampleTime=-1
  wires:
  In1/1 -> To Workspace/1

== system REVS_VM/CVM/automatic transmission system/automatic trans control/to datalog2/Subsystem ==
  In1 : Inport
  Enable : EnablePort
  To Workspace : ToWorkspace  VariableName=datalog__transmission__command_line_pressure_bar  SampleTime=-1
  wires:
  In1/1 -> To Workspace/1

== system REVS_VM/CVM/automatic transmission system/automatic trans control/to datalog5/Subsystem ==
  In1 : Inport
  Enable : EnablePort
  To Workspace : ToWorkspace  VariableName=datalog__transmission__current_gear  SampleTime=-1
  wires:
  In1/1 -> To Workspace/1

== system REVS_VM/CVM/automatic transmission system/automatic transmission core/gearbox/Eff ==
  Efficiency : Inport
  Input : Inport  Port=2
  Math Function : Math  Operator=reciprocal
  Product1 : Product
  Switch : Switch  ZeroCross=off
  Output : Outport
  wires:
  Math Function/1 -> Switch/3
  Product1/1 -> Output/1
  Input/1 -> Product1/2, Switch/2
  Efficiency/1 -> Switch/1, Math Function/1
  Switch/1 -> Product1/1

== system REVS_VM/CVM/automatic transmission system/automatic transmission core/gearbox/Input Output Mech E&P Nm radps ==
  trq_in_Nm : Inport
  spd_in_radps : Inport  Port=2
  iner_in_kgm2 : Inport  Port=3
  trq_out_Nm : Inport  Port=4
  spd_out_radps : Inport  Port=5
  iner_out_kgm2 : Inport  Port=6
  Compare To Constant : simulink/Logic and Bit Operations/Compare To Constant  relop=>=  const=1  OutDataTypeStr=boolean
  Constant : Constant  Value=VerboseSignal
  Subsystem : Subsystem
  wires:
  trq_in_Nm/1 -> Subsystem/1(trq_in_Nm)
  spd_in_radps/1 -> Subsystem/2(spd_in_radps)
  iner_in_kgm2/1 -> Subsystem/3(iner_in_kgm2)
  trq_out_Nm/1 -> Subsystem/4(trq_out_Nm)
  spd_out_radps/1 -> Subsystem/5(spd_out_radps)
  iner_out_kgm2/1 -> Subsystem/6(iner_out_kgm2)
  Compare To Constant/1 -> Subsystem/Enable
  Constant/1 -> Compare To Constant/1

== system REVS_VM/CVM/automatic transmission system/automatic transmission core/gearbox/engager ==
  tgt_gear_num : Inport
  Compare To Constant1 : simulink/Logic and Bit Operations/Compare To Constant  relop=>  const=0  OutDataTypeStr=boolean  ZeroCross=off
  Compare To Constant2 : simulink/Logic and Bit Operations/Compare To Constant  relop=~=  const=0  OutDataTypeStr=boolean
  Compare To Constant3 : simulink/Logic and Bit Operations/Compare To Constant  relop=>=  const=1  OutDataTypeStr=boolean  ZeroCross=off
  Compare To Constant4 : simulink/Logic and Bit Operations/Compare To Constant  relop=~=  const=1  OutDataTypeStr=boolean  ZeroCross=off
  Compare To Constant5 : simulink/Logic and Bit Operations/Compare To Constant  relop=~=  const=0  OutDataTypeStr=boolean
  Constant1 : Constant  Value=gear.number
  Constant2 : Constant  Value=gear.type == enum_transmission_type.CVT
  Data Type Conversion : DataTypeConversion  OutDataTypeStr=double
  IC : InitialCondition  Value=0
  Logical Operator : Logic  Operator=OR  AllPortsSameDT=off  OutDataTypeStr=boolean
  Logical Operator1 : Logic  Operator=OR  Inputs=1  AllPortsSameDT=off  OutDataTypeStr=boolean
  Logical Operator2 : Logic  Inputs=3  AllPortsSameDT=off  OutDataTypeStr=boolean
  Memory1 : Memory  X0=gear.number(2)
  Memory2 : Memory  X0=gear.number(2)
  Product : Product
  Product1 : Product
  Rate Limiter : RateLimiter  RisingSlewLimit=1/gear.shift_duration_secs  FallingSlewLimit=-inf  InitialCondition=1
  Relational Operator : RelationalOperator  Operator===  OutDataTypeStr=boolean
  Relational Operator2 : RelationalOperator  Operator===  OutDataTypeStr=boolean
  Saturation : Saturate  UpperLimit=1  LowerLimit=0  ZeroCross=off
  Saturation1 : Saturate  UpperLimit=1 - 0.10 * (gear.type == enum_transmission_type.CVT)  LowerLimit=eps + 0.89 * (gear.type == enum_transmission_type.CVT)  ZeroCross=off
  Switch : Switch  Criteria=u2 > Threshold
  Switch1 : Switch  Criteria=u2 > Threshold
  to datalog with base name : Subsystem
  to datalog with base name1 : Subsystem
  to datalog with base name2 : Subsystem
  engage : Outport
  curr_gear_num : Outport  Port=2
  cmd_gear_num : Outport  Port=3
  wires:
  Logical Operator1/1 -> Logical Operator/1
  Constant2/1 -> Logical Operator/2
  Compare To Constant1/1 -> Product1/1
  Switch1/1 -> Product1/2
  Memory1/1 -> Switch1/3
  Rate Limiter/1 -> Saturation/1
  Data Type Conversion/1 -> Saturation1/1
  Compare To Constant2/1 -> Product/1
  Memory2/1 -> cmd_gear_num/1, Switch/3, to datalog with base name2/1(Var), Relational Operator/2, Switch1/1
  IC/1 -> Rate Limiter/1
  Product/1 -> IC/1
  Relational Operator/1 -> Data Type Conversion/1
  Switch/1 -> Memory2/1
  Saturation/1 -> to datalog with base name1/1(Var), Compare To Constant3/1, Compare To Constant4/1, Compare To Constant1/1, engage/1
  Saturation1/1 -> Product/2
  tgt_gear_num/1 -> Relational Operator/1, Relational Operator2/1, Compare To Constant5/1, Switch/1, Compare To Constant2/1
  Compare To Constant4/1 -> Logical Operator2/1
  Product1/1 -> Memory1/1, to datalog with base name/1(Var), curr_gear_num/1
  Compare To Constant3/1 -> Switch1/2
  Constant1/1 -> Relational Operator2/2
  Relational Operator2/1 -> Logical Operator1/1
  Compare To Constant5/1 -> Logical Operator2/2
  Logical Operator/1 -> Logical Operator2/3
  Logical Operator2/1 -> Switch/2

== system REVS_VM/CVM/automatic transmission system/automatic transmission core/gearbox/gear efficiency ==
  bus : Inport
  Bus Selector : BusSelector  OutputSignals=gb.gb_cmd_gear,gb_spd_in_radps,ctrl.gb_line_press_bar
  Lookup : Lookup_n-D  NumberOfTableDimensions=10  BreakpointsForDimension1=LookupStructure.axis_1.breakpoints  BreakpointsForDimension2=LookupStructure.axis_2.breakpoints  BreakpointsForDimension3=LookupStructure.axis_3.breakpoints  BreakpointsForDimension4=LookupStructure.axis_4.breakpoints  BreakpointsForDimension5=LookupStructure.axis_5.breakpoints  BreakpointsForDimension6=LookupStructure.axis_6.breakpoints  BreakpointsForDimension7=LookupStructure.axis_7.breakpoints  BreakpointsForDimension8=LookupStructure.axis_8.breakpoints  BreakpointsForDimension9=LookupStructure.axis_9.breakpoints  BreakpointsForDimension10=LookupStructure.axis_10.breakpoints  IndexSearchMethod=Linear search  BeginIndexSearchUsingPreviousIndexResult=on  Table=LookupStructure.table  DiagnosticForOutOfRangeInput=Warning  InternalRulePriority=Speed  RndMeth=Simplest  SupportTunableTableSize=on  MaximumIndicesForEachDimension=LookupStructure.table_size
  out : Outport
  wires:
  bus/1 -> Bus Selector/1
  Lookup/1 -> out/1
